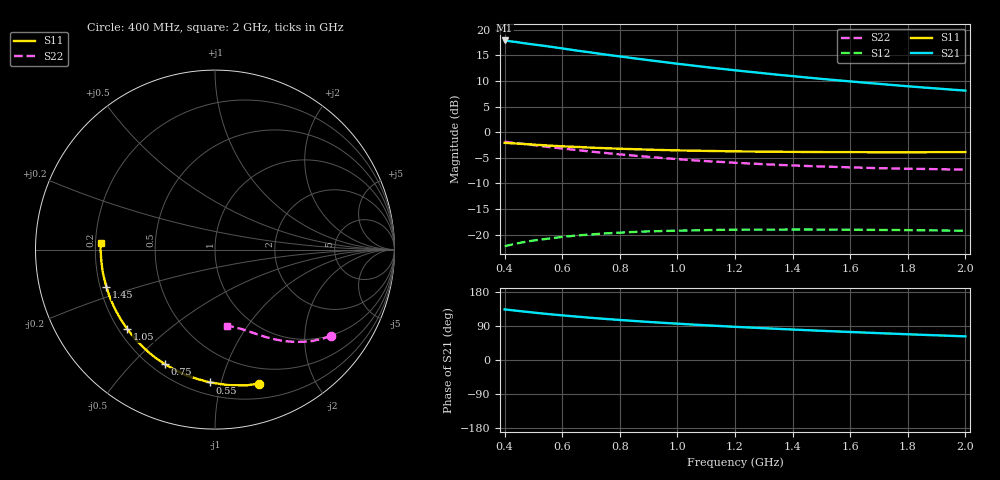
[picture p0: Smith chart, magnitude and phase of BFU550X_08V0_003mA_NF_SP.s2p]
! Filename:  P:\Prog\Test\Noise\ATS_data\Testdata_Net\BFU550X no attenuator noise\BFU550X_APG2013_44_C05_08p0V_003mA_NF_CM01_D.sf
! Date/Time: Fri 26/Jul/2013 14:37:13
! BFU550X_APG2013_44_C05_08p0V_1to10mA_NF_CM01_Bias3_R.sf
! Noise Parameter Data File
! BFU550X_APG2013_44_C05_08p0V_1to10mA_NF_CM01
! Date/time: Wed Jul 24 17:16:38 2013
! VAR V_out= 8.000000
! VAR I_out= 3.000000
! VAR V_in= 0.798000
! VAR I_in= 0.031705
! Device data file deembeded for feedlines and parallel
! Original file: \BFU550X no attenuator noise\BFU550X_APG2013_44_C05_08p0V_003mA_NF_CM01_R.sf
! Feed-files: PR005V01_100713_Feed1.s2p, PR005V01_100713_Feed2.s2p
! Parallel-file: PR005V01_100713_Par.s2p
# MHz S MA R 50
!  Freq-MHz  S11-mag  S11-arg  S21-mag  S21-arg  S12-mag  S12-arg  S22-mag  S22-arg
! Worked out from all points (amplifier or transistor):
!   37 points, 400 MHz to 2 GHz, reference 50 ohm
!   highest |S21| = 17.9 dB at 400 MHz (marker M1)
!   |S21| within 3 dB of that: start of sweep to 784.2 MHz
!   unconditionally stable (mu >= 1): nowhere
!   at 500 MHz: K = 0.19, MSG = 19.1 dB, |S12| = -21.2 dB
!   at 1.1 GHz: K = 0.41, MSG = 15.9 dB, |S12| = -19.1 dB
!   at 2 GHz: K = 0.75, MSG = 13.7 dB, |S12| = -19.2 dB
!   lowest NFmin = 0.58 dB at 420 MHz
!   S11 on the Smith chart (normalised r, x): 400 MHz: 0.34, -1.33; 550 MHz: 0.28, -0.92; 750 MHz: 0.25, -0.63; 1.05 GHz: 0.23, -0.37; 1.45 GHz: 0.23, -0.16; 2 GHz: 0.22, +0.03
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400  0.7866 -71.8  7.847 133.6  0.07706 51.5  0.8073 -36.7
420  0.7795 -74.6  7.698 131.8  0.07929 50.2  0.7923 -38.1
440  0.7741 -77.6  7.583 130.2  0.08166 48.9  0.7826 -39.2
480  0.7623 -82.9  7.292 126.9  0.08557 46.4  0.7571 -41.7
550  0.7405 -92.2  6.874 121.3  0.09121 42.3  0.7177 -45.6
600  0.727 -98.1  6.566 117.8  0.09481 39.8  0.6922 -48.0
650  0.7173 -103.5  6.253 114.5  0.09796 37.5  0.6689 -50.1
700  0.7055 -108.8  5.988 111.3  0.1003 35.4  0.6456 -52.2
750  0.6968 -113.6  5.715 108.5  0.1026 33.6  0.626 -54.0
800  0.689 -118.3  5.483 105.6  0.1044 31.8  0.6062 -55.8
850  0.6815 -122.7  5.253 103.0  0.1061 30.2  0.5894 -57.4
900  0.6742 -126.9  5.042 100.5  0.1074 28.7  0.5738 -58.9
950  0.6687 -130.8  4.841 98.1  0.1083 27.4  0.5578 -60.4
1050  0.6594 -137.8  4.477 93.7  0.1098 25.1  0.5319 -63.0
1100  0.6555 -141.2  4.31 91.6  0.1105 24.1  0.5211 -64.1
1200  0.6492 -147.4  4.015 87.6  0.1115 22.2  0.5021 -66.4
1300  0.6449 -153.1  3.754 83.9  0.1119 20.7  0.4863 -68.5
1450  0.64 -160.8  3.412 78.7  0.112 18.9  0.4671 -71.4
1500  0.6389 -163.2  3.308 77.1  0.1119 18.3  0.4618 -72.4
1600  0.6381 -167.8  3.126 73.9  0.1115 17.5  0.4528 -74.3
1750  0.6362 -174.1  2.879 69.4  0.1108 16.5  0.4418 -76.9
2000  0.6386 176.5  2.542 62.4  0.1091 15.9  0.4311 -81.1
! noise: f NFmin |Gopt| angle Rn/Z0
400  0.6093  0.3313  29.35  0.1545
460  0.6141  0.3026  44.13  0.1214
600  0.6982  0.3272  49.74  0.1431
800  0.7025  0.348  71.07  0.1175
1000  0.7707  0.3529  85.36  0.1089
1200  0.7821  0.3783  100.7  0.1022
1400  0.8657  0.3958  113.6  0.0904
1600  0.8246  0.4158  129.5  0.0717
1800  0.8829  0.4406  144.8  0.0561
2000  0.9478  0.5187  154.6  0.0416
